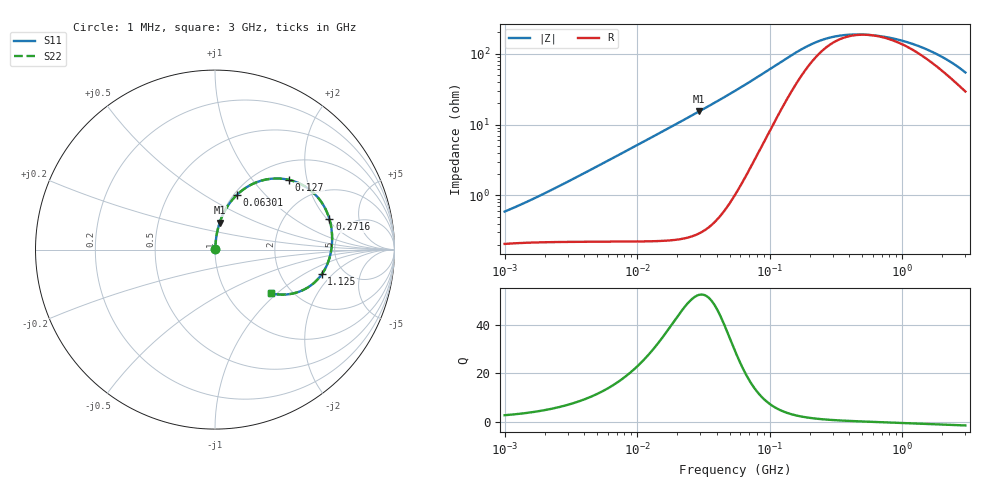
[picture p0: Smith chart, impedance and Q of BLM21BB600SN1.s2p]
! BLM21BB600SN1
# Hz S RI R 50
!Freq.(Hz) S11(Real) S11(Imag) S21(Real) S21(Imag) S12(Real) S12(Imag) S22(Real) S22(Imag)
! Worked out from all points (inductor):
!   401 points, 1 MHz to 3 GHz, reference 50 ohm
!   read as one part in series: L = 84.7 nH near 1.174 MHz
!   highest Q = 52.6 at 29.45 MHz (marker M1), where L = 83 nH
!   self-resonance near 554.3 MHz
!   S11 on the Smith chart (normalised r, x): 1 MHz: 1.00, +0.01; 63.01 MHz: 1.03, +0.70; 127 MHz: 1.37, +1.57; 271.6 MHz: 3.51, +2.13; 1.125 GHz: 3.43, -1.50; 3 GHz: 1.59, -0.92
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1000000  0.0021 0.00552  0.9979 -0.00552  0.9979 -0.00552  0.0021 0.00552
1716745  0.00225 0.009  0.9978 -0.009  0.9978 -0.009  0.00225 0.009
3823119  0.0026 0.0196  0.9974 -0.0196  0.9974 -0.0196  0.0026 0.0196
1.461624e7  0.00783 0.0743  0.9922 -0.0743  0.9922 -0.0743  0.00783 0.0743
2.944989e7  0.0257 0.1492  0.9743 -0.1492  0.9743 -0.1492  0.0257 0.1492
5.477226e7  0.0896 0.269  0.9104 -0.269  0.9104 -0.269  0.0896 0.269
6.301011e7  0.1198 0.3028  0.8802 -0.3028  0.8802 -0.3028  0.1198 0.3028
7.697298e7  0.1799 0.3497  0.8201 -0.3497  0.8201 -0.3497  0.1799 0.3497
9.402997e7  0.2624 0.3854  0.7376 -0.3854  0.7376 -0.3854  0.2624 0.3854
1.269575e8  0.4133 0.3882  0.5867 -0.3882  0.5867 -0.3882  0.4133 0.3882
1.646891e8  0.5302 0.3317  0.4698 -0.3317  0.4698 -0.3317  0.5302 0.3317
2.094008e8  0.5999 0.2541  0.4001 -0.2541  0.4001 -0.2541  0.5999 0.2541
2.716345e8  0.6374 0.1708  0.3626 -0.1708  0.3626 -0.1708  0.6374 0.1708
3.453811e8  0.6504 0.1048  0.3496 -0.1048  0.3496 -0.1048  0.6504 0.1048
4.480278e8  0.6523 0.0442  0.3477 -0.0442  0.3477 -0.0442  0.6523 0.0442
5.929311e8  0.6458 -0.0134  0.3542 0.0134  0.3542 0.0134  0.6458 -0.0134
8.005644e8  0.6297 -0.0717  0.3703 0.0717  0.3703 0.0717  0.6297 -0.0717
1.125055e9  0.595 -0.1375  0.405 0.1375  0.405 0.1375  0.595 -0.1375
1.519029e9  0.5421 -0.1935  0.4579 0.1935  0.4579 0.1935  0.5421 -0.1935
1.970482e9  0.4728 -0.2329  0.5272 0.2329  0.5272 0.2329  0.4728 -0.2329
2.455801e9  0.3953 -0.2501  0.6047 0.2501  0.6047 0.2501  0.3953 -0.2501
3e9  0.3125 -0.2434  0.6875 0.2434  0.6875 0.2434  0.3125 -0.2434
